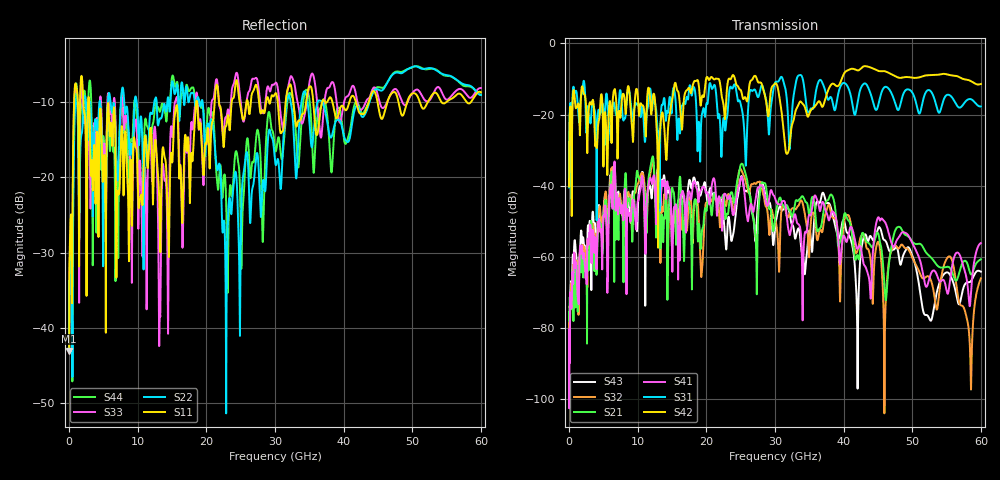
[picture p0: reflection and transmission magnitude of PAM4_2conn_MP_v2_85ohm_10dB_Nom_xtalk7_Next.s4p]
! Info: Touchstone file created by Circ.  Input file=FAB50GbE_2conn_Midplane_Examax_Topo2_v2_85ohm_10dB_Nom.circ
# Hz S RI R 50
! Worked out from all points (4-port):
!   6000 points, 10 MHz to 60 GHz, reference 50 ohm
!   strongest paths, dB at 10 MHz, 15.01 GHz, 30.01 GHz, 45.01 GHz, 60 GHz:
!     S42: -40.2, -15.9, -11.3, -7.7, -11.4
!     S31: -40.5, -17.1, -11.1, -17.6, -17.7
!     S41: -87.9, -59.6, -43.5, -49.0, -56.1
!     S21: -75.6, -40.6, -49.5, -53.3, -60.7
!     S32: -82.5, -48.8, -49.4, -55.8, -66.1
!     S43: -77.3, -56.4, -51.8, -52.2, -64.2
!   lowest |S11| = -43.1 dB at 10 MHz (marker M1), VSWR 1.01, Z = 50.7 + j0.0216 ohm
!   |S11| at or under -10 dB: 2.925 GHz to 18.53 GHz (15.61 GHz wide, 145 % of centre); 18.64 GHz to 21.21 GHz (2.572 GHz wide, 12.9 % of centre); 38.36 GHz to 40.85 GHz (2.486 GHz wide, 6.28 % of centre)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
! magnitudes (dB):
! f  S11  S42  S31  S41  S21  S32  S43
! 10 MHz  -43.1  -40.2  -40.5  -87.9  -75.6  -82.5  -77.3
! 990 MHz  -7.6  -18.2  -13.4  -61.7  -67.7  -63.9  -58.7
! 12.11 GHz  -18.0  -17.1  -18.7  -39.5  -32.2  -33.4  -42.1
! 19.31 GHz  -15.3  -15.6  -20.7  -40.9  -53.8  -64.9  -41.5
! 25.01 GHz  -10.8  -13.1  -17.1  -38.0  -34.1  -35.3  -37.8
! 42 GHz  -10.7  -7.6  -16.9  -57.8  -59.5  -58.4  -83.6
! 60 GHz  -8.7  -11.4  -17.7  -56.1  -60.7  -66.1  -64.2
